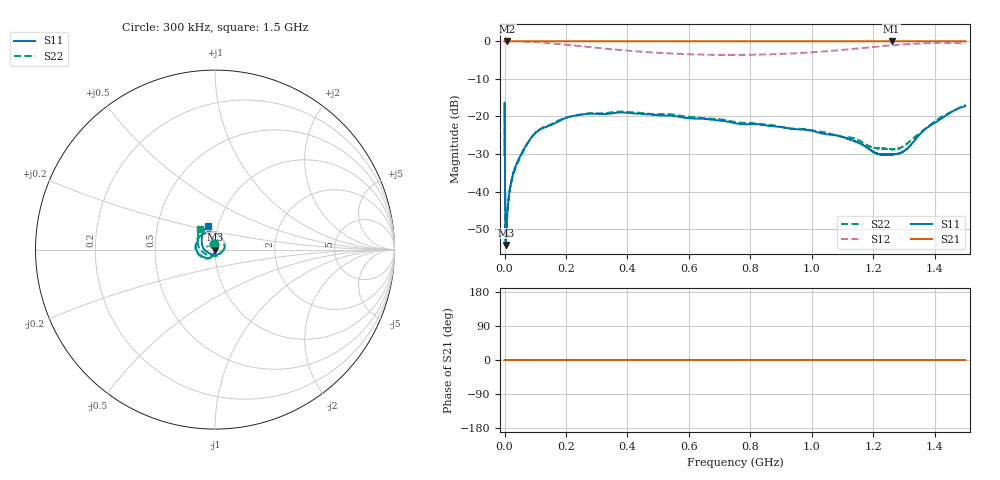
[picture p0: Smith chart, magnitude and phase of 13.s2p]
!Keysight Technologies,N5232A,MY52221221,A.10.65.11
!Date: Tuesday, May 21, 2024 18:50:10
!Correction: S11(Full 2 Port(1,4))
!S41(Full 2 Port(1,4))
!S14(Full 2 Port(1,4))
!S44(Full 2 Port(1,4))
!S2P File: Measurements: S11, S41, S14, S44:
# Hz S  RI  R 50
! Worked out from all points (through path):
!   16001 points, 300 kHz to 1.5 GHz, reference 50 ohm
!   highest |S21| = 0.02 dB at 1.26 GHz (marker M1); lowest = 0.0 dB at 9.017 MHz (marker M2)
!   lowest |S11| = -54.2 dB at 4.049 MHz (marker M3), VSWR 1.00, Z = 50.2 + j0.037 ohm
!   |S11| at or under -10 dB: start of sweep to end of sweep
!   |S22| runs from -54.5 to -16.3 dB; largest |S21 - S12| = 1.7
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300000  -0.00791 0.0294  0.9994 2.61e-05  0.3572 0.9614  -0.00403 0.0297
4049250  0.00191 0.000369  1 -5.1e-05  0.3344 0.9514  0.00184 -0.000363
9017006  0.00197 -0.00464  0.9993 0.000181  0.3477 0.9441  0.00177 -0.00464
1.032924e7  0.00186 -0.00577  0.9998 0.000652  0.3517 0.9428  0.00162 -0.0057
1.464088e7  0.00098 -0.00896  1 4.06e-05  0.3646 0.9375  0.000828 -0.00862
1.923371e7  -0.000308 -0.012  0.9999 0.000107  0.3792 0.931  -0.000416 -0.0116
3.216862e7  -0.00458 -0.0192  1.001 0.000178  0.4183 0.912  -0.00446 -0.0183
5.391428e7  -0.0119 -0.029  0.9998 -0.000213  0.4811 0.8743  -0.0111 -0.028
8.859484e7  -0.0278 -0.0452  1 0.000102  0.5686 0.8004  -0.0269 -0.0456
1.273996e8  -0.0528 -0.0466  0.9995 9.93e-05  0.6469 0.7075  -0.0522 -0.0491
2.502812e8  -0.1057 0.00219  1 0.0002  0.7563 0.4081  -0.1066 -0.00312
3.754125e8  -0.0894 0.0683  1.001 0.000439  0.7477 0.1685  -0.0967 0.0635
5.002625e8  -0.0442 0.0937  0.9998 -3.37e-05  0.7028 -0.00237  -0.0529 0.093
7.5015e8  0.0214 0.0784  1 0.000259  0.6074 -0.2502  0.0158 0.0828
1.000131e9  0.0534 0.036  1.001 0.00052  0.4992 -0.5085  0.0503 0.0417
1.144571e9  0.0459 -0.00309  1.001 0.000196  0.3765 -0.7041  0.0498 0.000346
1.21187e9  0.0221 -0.0232  1 0.000282  0.2774 -0.804  0.0318 -0.0204
1.250112e9  0.00699 -0.0304  1.001 0.00013  0.1925 -0.8547  0.0137 -0.0344
1.259673e9  0.00148 -0.0311  1.002 -0.000118  0.1721 -0.8632  0.00848 -0.0355
1.30457e9  -0.028 -0.022  1.001 0.00012  0.0603 -0.9116  -0.0182 -0.0376
1.370932e9  -0.0675 0.0113  1.001 -0.000335  -0.1329 -0.9332  -0.0679 -0.0134
1.5e9  -0.0372 0.1321  1.001 -0.000343  -0.5005 -0.7943  -0.0857 0.1136
